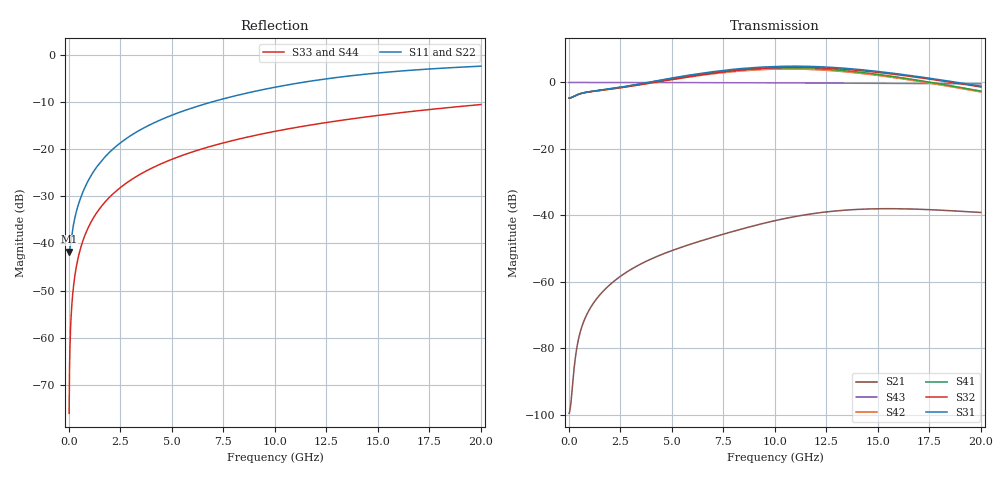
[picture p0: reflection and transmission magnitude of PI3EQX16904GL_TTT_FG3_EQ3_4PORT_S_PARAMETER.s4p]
! NPort=4 DATA=2000 NOISE=0 GROUPDELAY=0 COMPLEX_DATAFORMAT=POLAR
! NumOfBlock=1 NumOfParam=0
! .MODEL Smodel S TSTONEFILE=PI3EQX16904GL_TTT_FG3_EQ3_4PORT_S_PARAMETER.s4p TYPE=S
!  -- The above .MODEL line can be used for the S element in the netlist.
! The s parameter is extracted from the linear redriver, it is not bi-directional; only s(4,1)s(4,2) and s(3,1)s(3,2)
! should be the insertion loss
!Port definition:
!Port1 = input+
!Port2 = input-
!Port3 = output+
!Port4 = output-
# Hz S MA R  50
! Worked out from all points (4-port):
!   2000 points, 10 MHz to 20 GHz, reference 50 ohm
!   strongest paths, dB at 10 MHz, 5.01 GHz, 10.01 GHz, 15.01 GHz, 20 GHz:
!     S31: -4.7, 1.3, 4.8, 3.3, -1.1
!     S32: -4.7, 1.0, 4.4, 3.0, -1.4
!     S41: -4.7, 1.2, 4.4, 2.4, -2.6
!     S42: -4.7, 0.9, 4.0, 2.1, -2.9
!     S43: 0.0, 0.0, -0.1, -0.3, -0.4
!     S21: -99.6, -50.6, -41.6, -38.0, -39.1
!   lowest |S11| = -41.7 dB at 10 MHz (marker M1), VSWR 1.02, Z = 49.2 - j0.0603 ohm
!   |S11| at or under -10 dB: start of sweep to 6.902 GHz
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1e7  0.008182 -175.7  1.05e-05 7.6  0 0.0  0 0.0
     1.05e-05 7.6  0.008182 -175.7  0 0.0  0 0.0
     0.5834 0.2  0.5834 -179.8  0.0001571 -90.0  1 -0.0
     0.5834 -179.8  0.5834 0.2  1 -0.0  0.0001571 -90.0
3.9e8  0.02299 -119.3  0.0001042 117.3  0 0.0  0 0.0
       0.0001042 117.3  0.02299 -119.3  0 0.0  0 0.0
       0.65 5.8  0.6491 -174.5  0.006126 -90.4  1 -0.4
       0.6499 -174.9  0.649 4.8  1 -0.4  0.006126 -90.4
1.64e9  0.07788 -102.7  0.0007104 105.0  0 0.0  0 0.0
        0.0007104 105.0  0.07789 -102.7  0 0.0  0 0.0
        0.7741 -0.5  0.7679 178.5  0.02575 -91.5  0.9996 -1.5
        0.773 176.5  0.7669 -4.5  0.9996 -1.5  0.02575 -91.5
6.12e9  0.2806 -105.3  0.003894 81.8  0 0.0  0 0.0
        0.003871 81.8  0.2805 -105.4  0 0.0  0 0.0
        1.331 -40.5  1.267 138.8  0.09566 -95.7  0.995 -5.5
        1.306 128.6  1.244 -52.1  0.995 -5.5  0.09566 -95.7
9.93e9  0.4529 -112.8  0.008303 55.8  0 0.0  0 0.0
        0.008226 56.4  0.4521 -112.8  0 0.0  0 0.0
        1.738 -99.5  1.664 80.8  0.154 -99.2  0.9871 -8.9
        1.656 63.2  1.586 -116.4  0.9871 -8.9  0.154 -99.2
1.395e10  0.6122 -122.7  0.01234 14.2  0 0.0  0 0.0
          0.01227 15.1  0.6109 -122.7  0 0.0  0 0.0
          1.583 -167.5  1.528 13.1  0.2136 -102.8  0.975 -12.3
          1.446 -11.0  1.395 169.5  0.975 -12.3  0.2136 -102.8
2e10  0.763 -135.8  0.01113 -35.0  0 0.0  0 0.0
      0.01106 -33.9  0.7623 -135.7  0 0.0  0 0.0
      0.8804 106.6  0.8552 -72.9  0.2986 -108.1  0.9506 -17.4
      0.7413 -105.4  0.7201 75.2  0.9506 -17.4  0.2986 -108.1
